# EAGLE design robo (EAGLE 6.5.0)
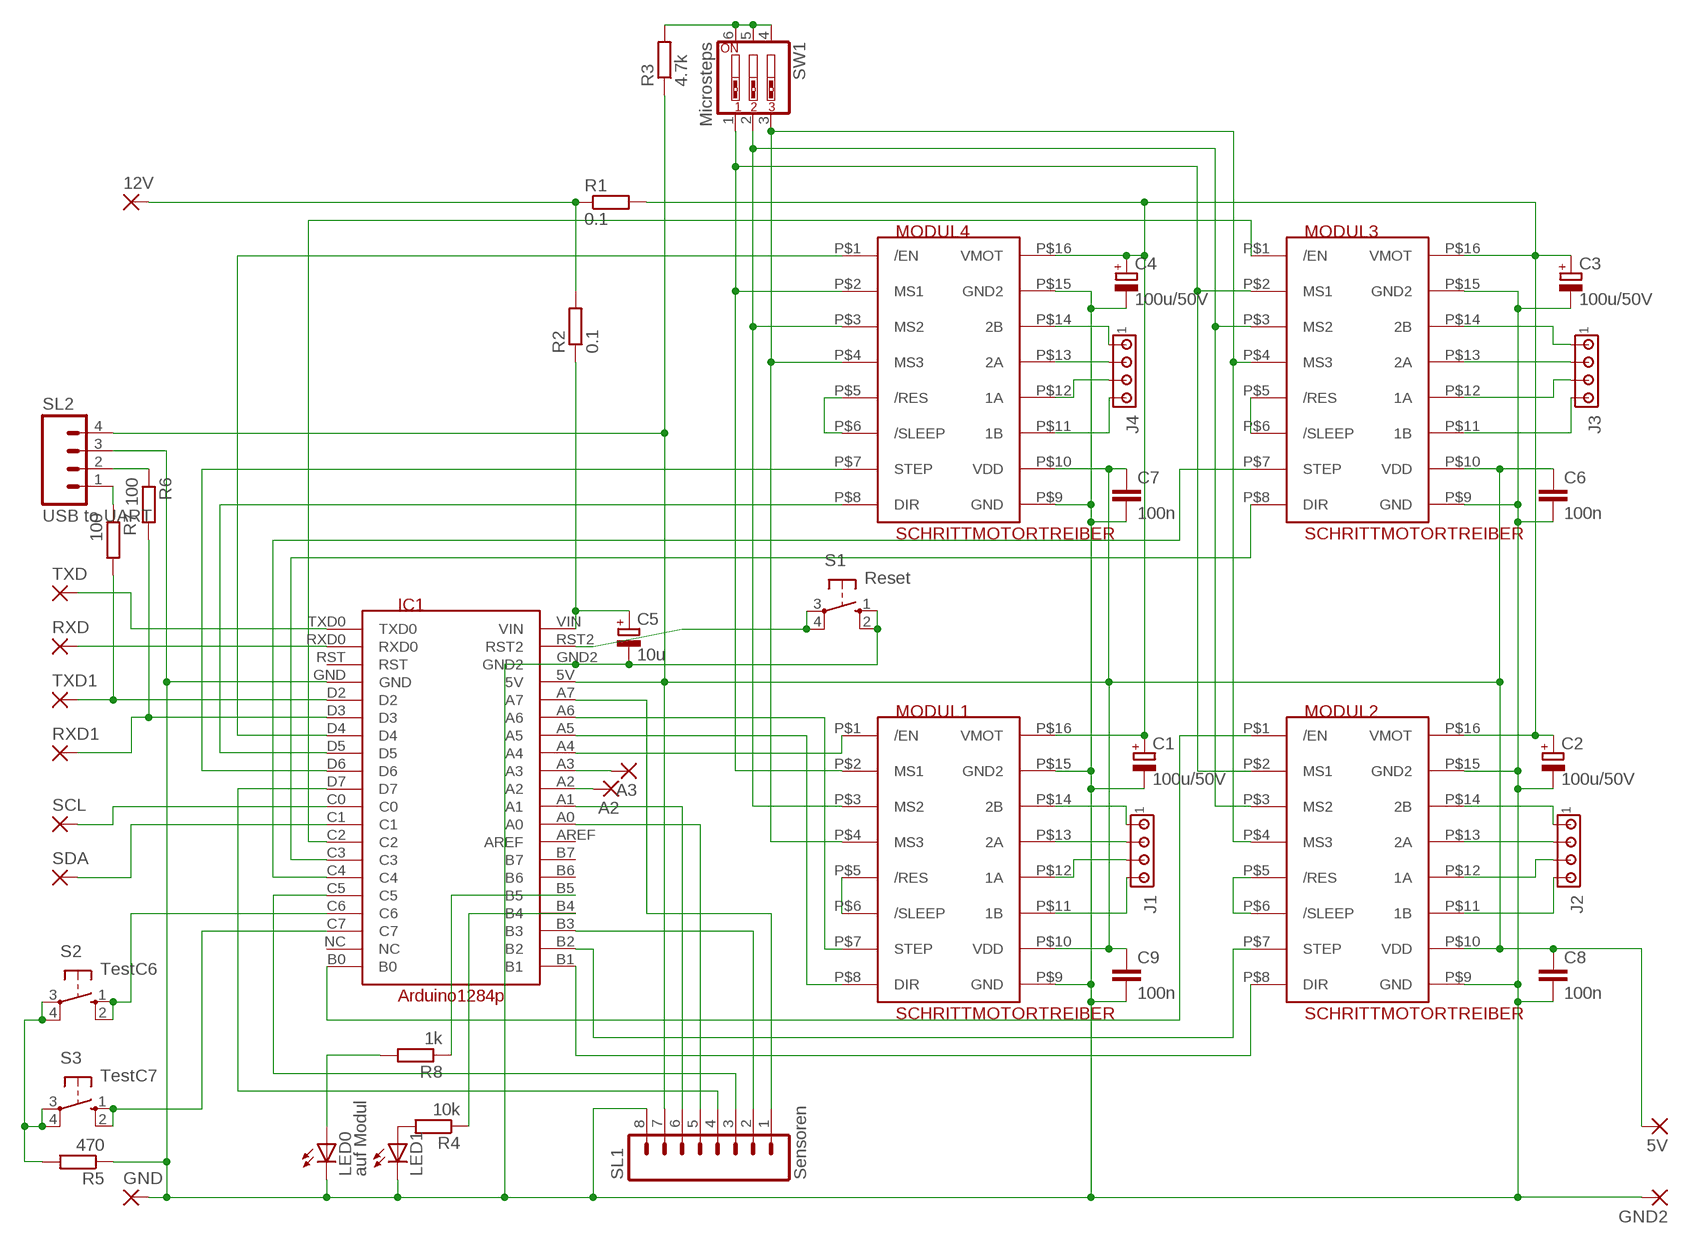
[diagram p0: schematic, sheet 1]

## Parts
5V  WIREPAD2,54/0,9  [2,54/0,9]
12V  WIREPAD3,17/1,1  [3,17/1,1]
A2  WIREPAD2,54/0,9  [2,54/0,9]
A3  WIREPAD2,54/0,9  [2,54/0,9]
C1  100u/50V  CPOL-EUE3.5-8  [E3,5-8]
C2  100u/50V  CPOL-EUE3.5-8  [E3,5-8]
C3  100u/50V  CPOL-EUE3.5-8  [E3,5-8]
C4  100u/50V  CPOL-EUE3.5-8  [E3,5-8]
C5  10u  CPOL-EUE2.5-6  [E2,5-6]
C6  100n  C2,5-3  [C2.5-3]
C7  100n  C2,5-3  [C2.5-3]
C8  100n  C2,5-3  [C2.5-3]
C9  100n  C2,5-3  [C2.5-3]
GND  WIREPAD3,17/1,1  [3,17/1,1]
GND2  WIREPAD2,54/0,9  [2,54/0,9]
IC1  Arduino1284p  ARDUINO1284P  [ARDUINO1284P]
J1  MTA04-100  [10X04MTA]
J2  MTA04-100  [10X04MTA]
J3  MTA04-100  [10X04MTA]
J4  MTA04-100  [10X04MTA]
LED0  auf Modul  LED3MM  [LED3MM]
LED1  LED3MM  [LED3MM]
MODUL1  SCHRITTMOTORTREIBER  [SCHRITTMOTORTREIBER]
MODUL2  SCHRITTMOTORTREIBER  [SCHRITTMOTORTREIBER]
MODUL3  SCHRITTMOTORTREIBER  [SCHRITTMOTORTREIBER]
MODUL4  SCHRITTMOTORTREIBER  [SCHRITTMOTORTREIBER]
R1  0.1  R-EU_0204/7  [0204/7]
R2  0.1  R-EU_0204/7  [0204/7]
R3  4.7k  R-EU_0204/7  [0204/7]
R4  10k  R-EU_0204/7  [0204/7]
R5  470  R-EU_0204/7  [0204/7]
R6  100  R-EU_0207/12  [0207/12]
R7  100  R-EU_0207/12  [0207/12]
R8  1k  R-EU_0204/7  [0204/7]
RXD  WIREPAD2,54/0,9  [2,54/0,9]
RXD1  WIREPAD2,54/0,9  [2,54/0,9]
S1  Reset  10-XX  [B3F-10XX]
S2  TestC6  10-XX  [B3F-10XX]
S3  TestC7  10-XX  [B3F-10XX]
SCL  WIREPAD2,54/0,9  [2,54/0,9]
SDA  WIREPAD2,54/0,9  [2,54/0,9]
SL1  Sensoren  M08  [08P]
SL2  USB to UART  M04  [04P]
SW1  Microsteps  SW_DIP-3  [EDG-03]
TXD  WIREPAD2,54/0,9  [2,54/0,9]
TXD1  WIREPAD2,54/0,9  [2,54/0,9]

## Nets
GND [sehrdick]: C1.- C2.- C3.- C4.- C5.- C6.2 C7.2 C8.2 C9.2 GND2.1(P) GND.1(P) IC1.GND IC1.GND2 LED0.K(C) LED1.K(C) MODUL1.P$9(GND) MODUL1.P$15(GND2) MODUL2.P$9(GND) MODUL2.P$15(GND2) MODUL3.P$9(GND) MODUL3.P$15(GND2) MODUL4.P$9(GND) MODUL4.P$15(GND2) R5.1 S1.1(S) S1.2(S1) SL1.8 SL2.3
N$1 [dick]: J3.1 MODUL3.P$14(2B)
N$2 [dick]: J3.2 MODUL3.P$13(2A)
N$3 [dick]: J3.4 MODUL3.P$11(1B)
N$4: MODUL4.P$5(/RES) MODUL4.P$6(/SLEEP)
N$5: MODUL3.P$5(/RES) MODUL3.P$6(/SLEEP)
N$6: MODUL2.P$5(/RES) MODUL2.P$6(/SLEEP)
N$7: MODUL1.P$5(/RES) MODUL1.P$6(/SLEEP)
N$8 [dick]: J3.3 MODUL3.P$12(1A)
N$9 [dick]: J4.1 MODUL4.P$14(2B)
N$10 [dick]: J4.2 MODUL4.P$13(2A)
N$11 [dick]: J4.4 MODUL4.P$11(1B)
N$12 [dick]: J4.3 MODUL4.P$12(1A)
N$13 [dick]: J1.1 MODUL1.P$14(2B)
N$14 [dick]: J1.2 MODUL1.P$13(2A)
N$15 [dick]: J1.3 MODUL1.P$12(1A)
N$16 [dick]: J1.4 MODUL1.P$11(1B)
N$17 [dick]: J2.1 MODUL2.P$14(2B)
N$18 [dick]: J2.2 MODUL2.P$13(2A)
N$19 [dick]: J2.3 MODUL2.P$12(1A)
N$20 [dick]: J2.4 MODUL2.P$11(1B)
N$21 [sehrdick]: 12V.1(P) R1.1 R2.2
N$22: IC1.A0 SL1.5
N$23: IC1.A5 MODUL1.P$8(DIR)
N$24 [dick]: IC1.RXD0 RXD.1(P)
N$25: MODUL1.P$3(MS2) MODUL2.P$3(MS2) MODUL3.P$3(MS2) MODUL4.P$3(MS2) SW1.2
N$26 [dick]: IC1.TXD0 TXD.1(P)
N$27: MODUL1.P$4(MS3) MODUL2.P$4(MS3) MODUL3.P$4(MS3) MODUL4.P$4(MS3) SW1.3
N$28: R3.2 SW1.4 SW1.5 SW1.6
N$29: MODUL1.P$2(MS1) MODUL2.P$2(MS1) MODUL3.P$2(MS1) MODUL4.P$2(MS1) SW1.1
N$30: IC1.A6 MODUL1.P$7(STEP)
N$31: IC1.A7 SL1.1
N$32: IC1.A4 MODUL1.P$1(/EN)
N$33: IC1.B0 MODUL2.P$1(/EN)
N$34: IC1.B1 MODUL2.P$8(DIR)
N$35: IC1.B2 MODUL2.P$7(STEP)
N$36: IC1.B3 SL1.2
N$37: IC1.C2 MODUL3.P$1(/EN)
N$38: IC1.C3 MODUL3.P$8(DIR)
N$39: IC1.C4 MODUL3.P$7(STEP)
N$40: IC1.C5 SL1.3
N$41: IC1.D4 MODUL4.P$1(/EN)
N$42: IC1.D5 MODUL4.P$8(DIR)
N$43: IC1.D6 MODUL4.P$7(STEP)
N$44: IC1.D7 SL1.4
N$45 [dick]: IC1.D2 R7.2 TXD1.1(P)
N$46 [dick]: IC1.D3 R6.2 RXD1.1(P)
N$47: IC1.A1 SL1.6
N$48: IC1.RST2 S1.3(P) S1.4(P1)
N$49: IC1.C0 SCL.1(P)
N$50: IC1.C1 SDA.1(P)
N$51: A2.1(P) IC1.A2
N$52: A3.1(P) IC1.A3
N$53: LED1.A R4.2
N$54: IC1.B4 R4.1
N$55: IC1.C6 S2.1(S) S2.2(S1)
N$56: IC1.C7 S3.1(S) S3.2(S1)
N$57: R5.2 S2.3(P) S2.4(P1) S3.3(P) S3.4(P1)
N$58 [dick]: R7.1 SL2.1
N$59 [dick]: R6.1 SL2.2
N$60: LED0.A R8.2
N$61: IC1.B5 R8.1
VDD [dick]: 5V.1(P) C6.1 C7.1 C8.1 C9.1 IC1.5V MODUL1.P$10(VDD) MODUL2.P$10(VDD) MODUL3.P$10(VDD) MODUL4.P$10(VDD) R3.1 SL1.7 SL2.4
VIN [dick]: C5.+ IC1.VIN R2.1
VMOT [sehrdick]: C1.+ C2.+ C3.+ C4.+ MODUL1.P$16(VMOT) MODUL2.P$16(VMOT) MODUL3.P$16(VMOT) MODUL4.P$16(VMOT) R1.2
Unconnected: IC1.AREF IC1.B6 IC1.B7 IC1.NC IC1.RST

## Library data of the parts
5V 12V A2 A3 GND GND2 RXD RXD1 SCL SDA TXD TXD1 = wirepad:WIREPAD: Wire PAD connect wire on PCB
C1-C5 = rcl:CPOL-EU: POLARIZED CAPACITOR, European symbol
C6-C9 = capacitor-wima:C: CAPACITOR
IC1 = arduino:ARDUINO1284P
J1-J4 = con-amp:MTA04-100: AMP connector
LED0 LED1 = led:LED: LED
MODUL1-MODUL4 = arduino:SCHRITTMOTORTREIBER
R1-R8 = rcl:R-EU_: RESISTOR, European symbol
S1-S3 = switch-omron:10-XX: OMRON SWITCH; MPN: B3F-1000; OC_FARNELL: 176432; OC_NEWARK: 36M3542
SL1 = con-amp-quick:M08: AMP QUICK CONNECTOR; OC_FARNELL: unknown; OC_NEWARK: unknown
SL2 = con-amp-quick:M04: AMP QUICK CONNECTOR; OC_FARNELL: unknown; OC_NEWARK: unknown
SW1 = special:SW_DIP-3: DIP SWITCH

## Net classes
0 default: width 0.508 mm
1 dick: width 0.762 mm
2 sehrdick: width 1.27 mm

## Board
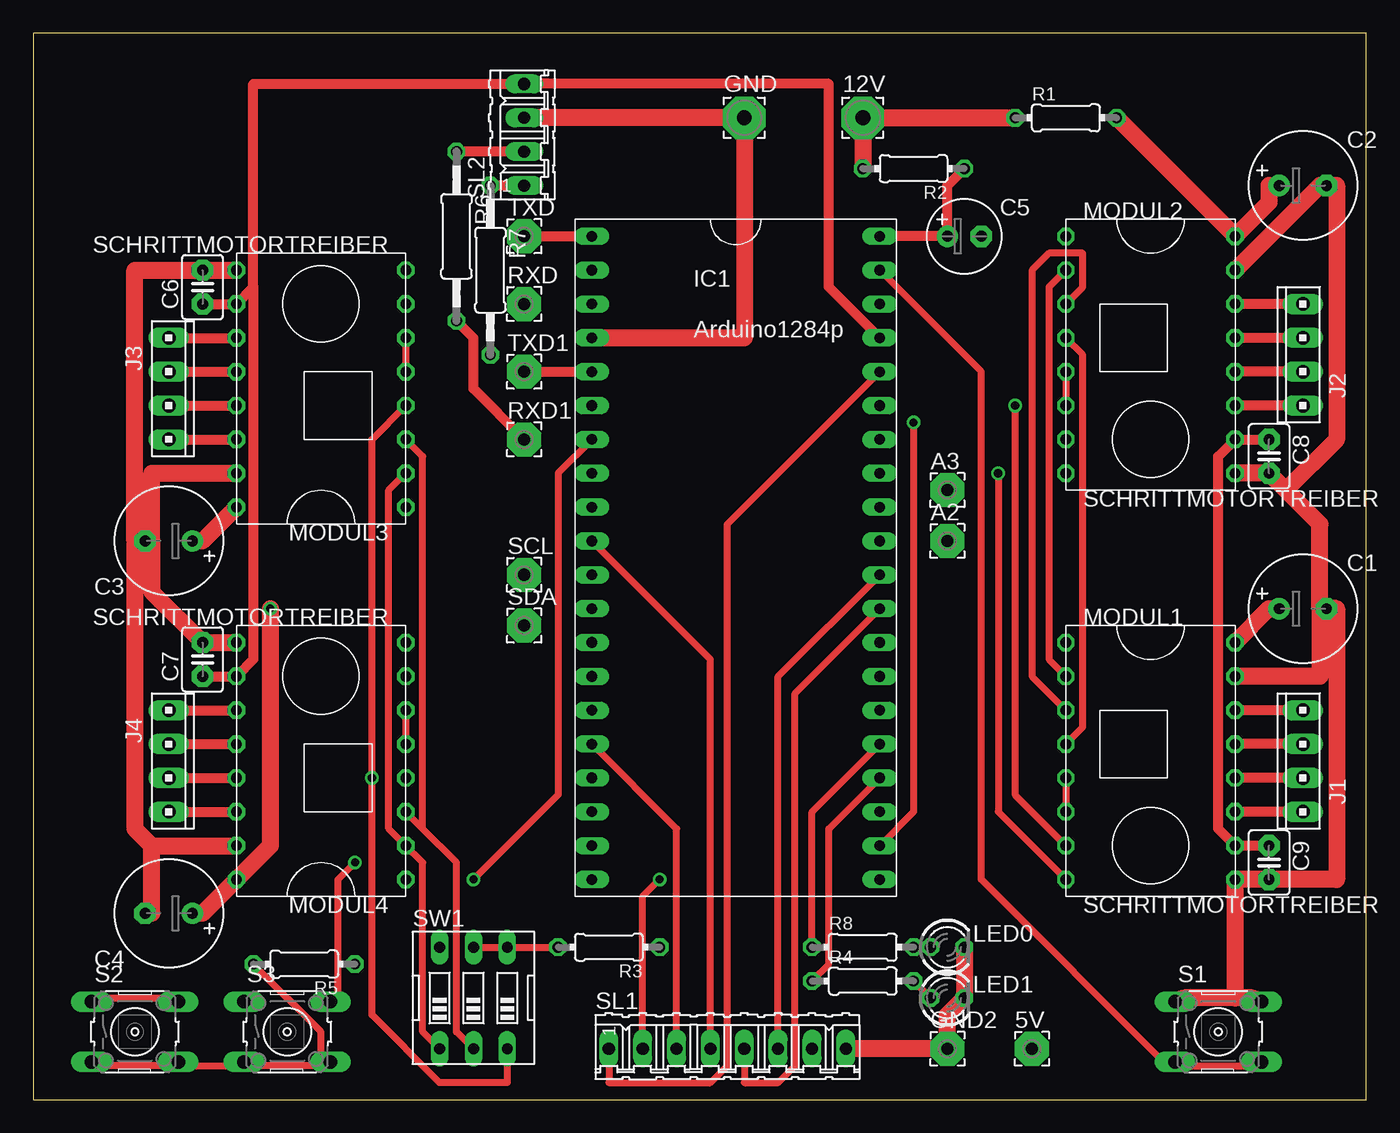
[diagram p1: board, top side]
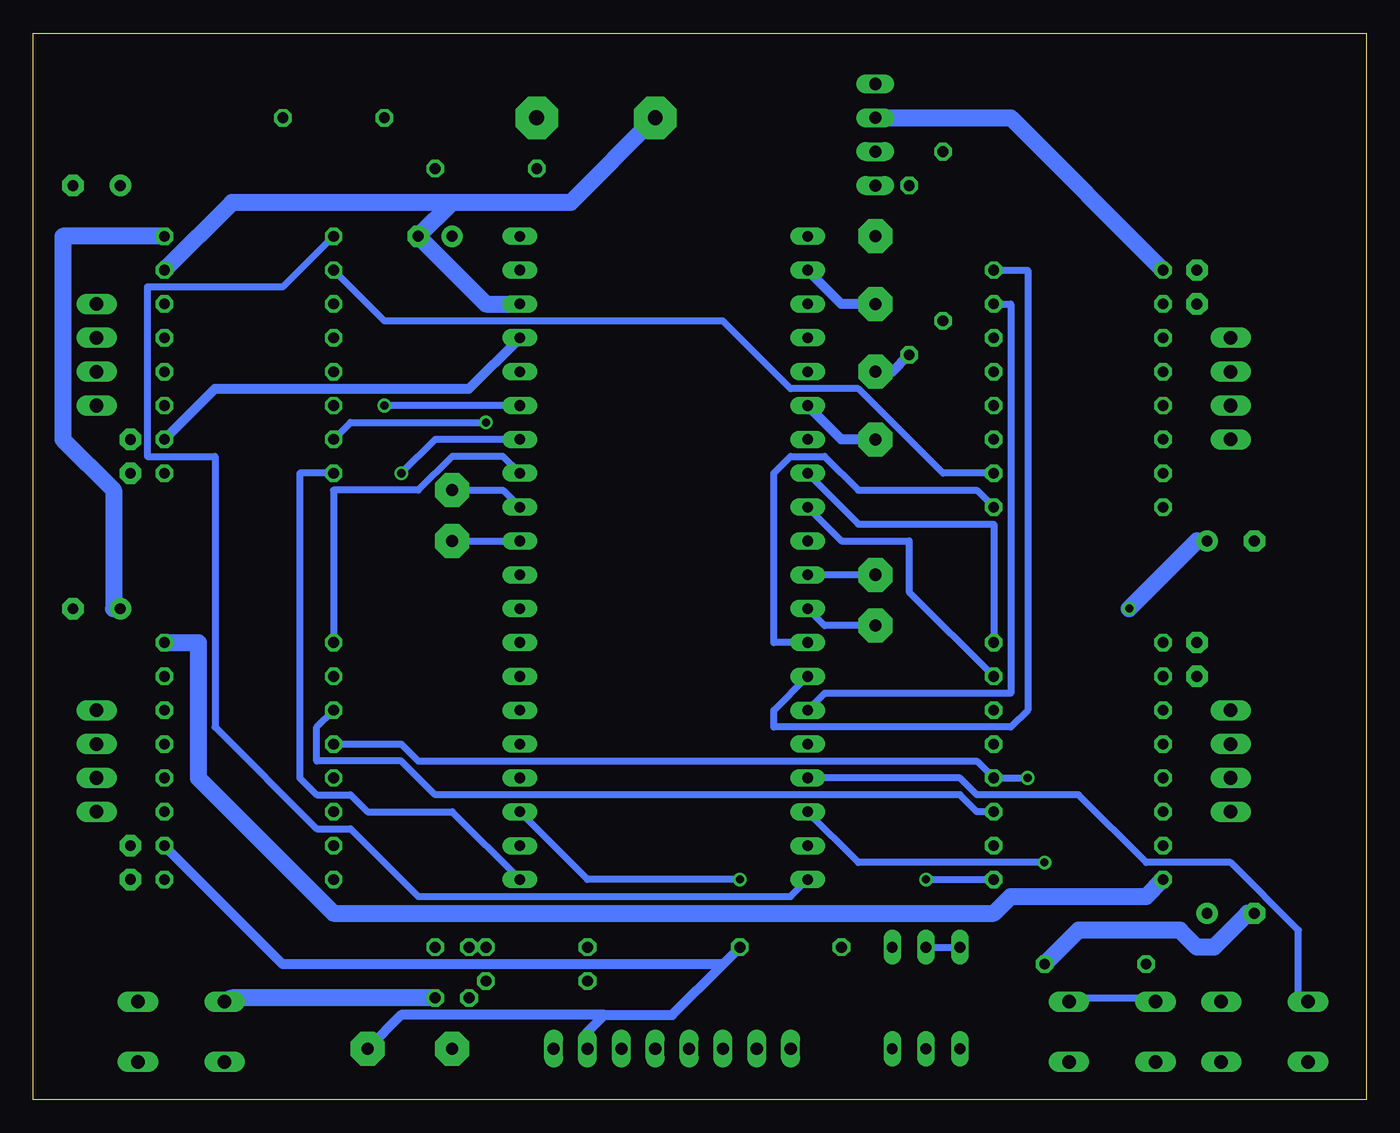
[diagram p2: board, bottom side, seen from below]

Size 100 x 80 mm. Coordinates in mm from the lower left corner, seen from the top.
Outline: 0,0 100,0 100,80 0,80 0,0
Copper layers (1*16): Top 0.035mm / dielectric 1.5mm / Bottom 0.035mm
Design rules "default": minimum track width 10mil, minimum drill 24mil, track to track 8mil, track to pad 8mil, pad to pad 8mil, via to via 8mil, smd to smd 8mil, copper to edge 40mil, drill to drill 8mil, minimum pad ring 10mil, minimum via ring 8mil, stop-mask expansion 4mil, vias tented up to drill 0mil, thermal gap 10mil

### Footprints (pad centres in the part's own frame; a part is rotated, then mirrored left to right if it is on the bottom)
2,54/0,9 = drill 0.914 pad 2.54 octagon: 1 0,0
3,17/1,1 = drill 1.118 pad 3.175 octagon: 1 0,0
E3,5-8 = drill 0.813 pad 1.6: + -1.778,0 | drill 0.813 pad 1.6 octagon: - 1.778,0
E2,5-6 = drill 0.813 pad 1.6: + -1.27,0 | drill 0.813 pad 1.6 octagon: - 1.27,0
C2.5-3 = drill 0.813 pad 1.6 octagon: 1 -1.27,0; 2 1.27,0
ARDUINO1284P = drill 0.8 long: 5V 10.16,3.81; A0 10.16,-16.51; A1 10.16,-13.97; A2 10.16,-11.43; A3 10.16,-8.89; A4 10.16,-6.35; A5 10.16,-3.81; A6 10.16,-1.27; A7 10.16,1.27; AREF 10.16,-19.05; B0 -11.43,-36.83; B1 10.16,-36.83; B2 10.16,-34.29; B3 10.16,-31.75; B4 10.16,-29.21; B5 10.16,-26.67; B6 10.16,-24.13; B7 10.16,-21.59; C0 -11.43,-13.97; C1 -11.43,-16.51; C2 -11.43,-19.05; C3 -11.43,-21.59; C4 -11.43,-24.13; C5 -11.43,-26.67; C6 -11.43,-29.21; C7 -11.43,-31.75; D2 -11.43,1.27; D3 -11.43,-1.27; D4 -11.43,-3.81; D5 -11.43,-6.35; D6 -11.43,-8.89; D7 -11.43,-11.43; GND -11.43,3.81; GND2 10.16,6.35; NC -11.43,-34.29; RST -11.43,6.35; RST2 10.16,8.89; RXD0 -11.43,8.89; TXD0 -11.43,11.43; VIN 10.16,11.43
10X04MTA = drill 1.016 long: 1 3.81,0; 2 1.27,0; 3 -1.27,0; 4 -3.81,0
LED3MM = drill 0.813 octagon: A -1.27,0; K 1.27,0
SCHRITTMOTORTREIBER = drill 0.8 octagon: P$1 -6.35,8.89; P$2 -6.35,6.35; P$3 -6.35,3.81; P$4 -6.35,1.27; P$5 -6.35,-1.27; P$6 -6.35,-3.81; P$7 -6.35,-6.35; P$8 -6.35,-8.89; P$9 6.35,-8.89; P$10 6.35,-6.35; P$11 6.35,-3.81; P$12 6.35,-1.27; P$13 6.35,1.27; P$14 6.35,3.81; P$15 6.35,6.35; P$16 6.35,8.89
0204/7 = drill 0.813 octagon: 1 -3.81,0; 2 3.81,0
0207/12 = drill 0.813 octagon: 1 -6.35,0; 2 6.35,0
B3F-10XX = drill 1.016 long: 1 -3.251,2.261; 2 3.251,2.261; 3 -3.251,-2.261; 4 3.251,-2.261
08P = drill 0.914 long: 1 -8.89,0; 2 -6.35,0; 3 -3.81,0; 4 -1.27,0; 5 1.27,0; 6 3.81,0; 7 6.35,0; 8 8.89,0
04P = drill 0.914 long: 1 -3.81,0; 2 -1.27,0; 3 1.27,0; 4 3.81,0
EDG-03 = drill 0.813 long: 1 -2.54,-3.81; 2 0,-3.81; 3 2.54,-3.81; 4 2.54,3.81; 5 0,3.81; 6 -2.54,3.81

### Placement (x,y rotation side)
5V  74.93,3.81 0 top
12V  62.23,73.66 0 top
A2  68.58,41.91 0 top
A3  68.58,45.72 0 top
C1  95.25,36.83 0 top
C2  95.25,68.58 0 top
C3  10.16,41.91 180 top
C4  10.16,13.97 180 top
C5  69.85,64.77 0 top
C6  12.7,60.96 90 top
C7  12.7,33.02 90 top
C8  92.71,48.26 270 top
C9  92.71,17.78 270 top
GND  53.34,73.66 0 top
GND2  68.58,3.81 0 top
IC1  53.34,53.34 0 top
J1  95.25,25.4 90 top
J2  95.25,55.88 90 top
J3  10.16,53.34 270 top
J4  10.16,25.4 270 top
LED0  68.58,11.43 0 top
LED1  68.58,7.62 0 top
MODUL1  83.82,25.4 0 top
MODUL2  83.82,55.88 0 top
MODUL3  21.59,53.34 180 top
MODUL4  21.59,25.4 180 top
R1  77.47,73.66 0 top
R2  66.04,69.85 180 top
R3  43.18,11.43 180 top
R4  62.23,8.89 0 top
R5  20.32,10.16 180 top
R6  31.75,64.77 270 top
R7  34.29,62.23 270 top
R8  62.23,11.43 0 top
RXD  36.83,59.69 0 top
RXD1  36.83,49.53 0 top
S1  88.9,5.08 0 top
S2  7.62,5.08 0 top
S3  19.05,5.08 0 top
SCL  36.83,39.37 0 top
SDA  36.83,35.56 0 top
SL1  52.07,3.81 0 top
SL2  36.83,72.39 90 top
SW1  33.02,7.62 0 top
TXD  36.83,64.77 0 top
TXD1  36.83,54.61 0 top

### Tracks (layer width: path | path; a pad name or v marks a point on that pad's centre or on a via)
GND
  Top 1.27: 8.89,19.05 MODUL4.P$15 | 8.89,19.05 8.89,13.97 C4.- | MODUL3.P$9 C6.2 7.62,62.23 7.62,41.91 | MODUL4.P$9 C7.2 8.89,38.1 8.89,41.91 | MODUL3.P$15 8.89,46.99 8.89,41.91 | 8.89,41.91 C3.- 7.62,41.91 | 8.89,19.05 7.62,20.32 7.62,41.91 | 90.17,7.62 91.44,7.62 S1.2 | 90.17,7.62 86.36,7.62 S1.1 | 90.17,7.62 MODUL1.P$9 C9.2 97.79,16.51 97.79,36.83 C1.- 96.52,36.83 | LED0.K LED1.K 68.58,6.35 GND2.1 SL1.8 | MODUL2.P$9 C8.2 93.98,45.72 | MODUL1.P$15 96.52,31.75 96.52,36.83 | 93.98,45.72 96.52,43.18 96.52,36.83 | MODUL2.P$15 96.52,68.58 C2.- 97.79,68.58 97.79,49.53 93.98,45.72 | IC1.GND 53.34,57.15 GND.1 SL2.3
  Bottom 1.27: R5.1 21.59,12.7 13.97,12.7 12.7,11.43 11.43,11.43 8.89,13.97 C4.- | LED1.K 85.09,7.62 S1.1 | IC1.GND2 66.04,59.69 C5.- 68.58,67.31 | 68.58,67.31 59.69,67.31 GND.1 | MODUL2.P$15 85.09,67.31 68.58,67.31 | MODUL3.P$9 26.67,73.66 SL2.3
N$1
  Top 0.762: J3.1 MODUL3.P$14
N$2
  Top 0.762: J3.2 MODUL3.P$13
N$3
  Top 0.762: J3.4 MODUL3.P$11
N$4
  Top 0.508: MODUL4.P$6 MODUL4.P$5
N$5
  Top 0.508: MODUL3.P$6 MODUL3.P$5
N$6
  Top 0.508: MODUL2.P$5 MODUL2.P$6
N$7
  Top 0.508: MODUL1.P$5 MODUL1.P$6
N$8
  Top 0.762: J3.3 MODUL3.P$12
N$9
  Top 0.762: J4.1 MODUL4.P$14
N$10
  Top 0.762: J4.2 MODUL4.P$13
N$11
  Top 0.762: J4.4 MODUL4.P$11
N$12
  Top 0.762: J4.3 MODUL4.P$12
N$13
  Top 0.762: J1.1 MODUL1.P$14
N$14
  Top 0.762: J1.2 MODUL1.P$13
N$15
  Top 0.762: J1.3 MODUL1.P$12
N$16
  Top 0.762: J1.4 MODUL1.P$11
N$17
  Top 0.762: J2.1 MODUL2.P$14
N$18
  Top 0.762: J2.2 MODUL2.P$13
N$19
  Top 0.762: J2.3 MODUL2.P$12
N$20
  Top 0.762: J2.4 MODUL2.P$11
N$21
  Top 1.27: R2.2 12V.1 R1.1
N$22
  Top 0.508: IC1.A0 57.15,30.48 57.15,2.54 55.88,1.27 53.34,1.27 SL1.5
N$23  (via drill 0.61)
  Top 0.508: MODUL1.P$8 72.39,21.59 v72.39,46.99
  Bottom 0.508: v72.39,46.99 69.85,49.53 IC1.A5
N$24
  Bottom 0.762: IC1.RXD0 39.37,59.69 RXD.1
N$25
  Top 0.508: MODUL1.P$3 74.93,31.75 74.93,62.23 76.2,63.5 78.74,63.5 78.74,60.96 MODUL2.P$3 | 29.21,20.32 31.75,17.78 31.75,5.08 SW1.2 | 29.21,20.32 MODUL4.P$3 | MODUL3.P$3 29.21,48.26 29.21,20.32
  Bottom 0.508: MODUL1.P$3 78.74,27.94 78.74,25.4 72.39,25.4 69.85,22.86 30.48,22.86 29.21,21.59 MODUL4.P$3
N$26
  Top 0.762: TXD.1 IC1.TXD0
N$27  (via drill 0.61)
  Top 0.508: MODUL3.P$4 25.4,49.53 v25.4,24.13 25.4,6.35 30.48,1.27 35.56,1.27 SW1.3 | MODUL2.P$4 78.74,55.88 78.74,27.94 MODUL1.P$4
  Bottom 0.508: MODUL1.P$4 72.39,26.67 71.12,25.4 29.21,25.4 MODUL4.P$4 v25.4,24.13
N$28
  Top 0.508: SW1.5 SW1.4 R3.2
  Bottom 0.508: SW1.5 SW1.6
N$29
  Top 0.508: MODUL1.P$2 76.2,33.02 76.2,60.96 MODUL2.P$2 | SW1.1 29.21,5.08 29.21,17.78 MODUL4.P$2 26.67,20.32 26.67,45.72 MODUL3.P$2
  Bottom 0.508: MODUL2.P$2 73.66,58.42 48.26,58.42 43.18,53.34 38.1,53.34 31.75,46.99 MODUL3.P$2
N$30  (via drill 0.61)
  Top 0.508: MODUL1.P$7 73.66,22.86 v73.66,52.07
  Bottom 0.508: IC1.A6 v73.66,52.07
N$31
  Top 0.508: IC1.A7 52.07,43.18 52.07,2.54 50.8,1.27 43.18,1.27 SL1.1
N$32
  Bottom 0.508: MODUL1.P$1 77.47,45.72 71.12,45.72 68.58,48.26 64.77,48.26 IC1.A4
N$33
  Bottom 0.508: IC1.B0 43.18,15.24 71.12,15.24 76.2,20.32 78.74,20.32 86.36,27.94 86.36,48.26 91.44,48.26 91.44,60.96 81.28,60.96 MODUL2.P$1
N$34
  Bottom 0.508: IC1.B1 68.58,21.59 74.93,21.59 76.2,22.86 78.74,22.86 80.01,24.13 80.01,46.99 MODUL2.P$8
N$35  (via drill 0.61)
  Top 0.508: IC1.B2 66.04,21.59 v66.04,50.8
  Bottom 0.508: v66.04,50.8 76.2,50.8 MODUL2.P$7
N$36  (via drill 0.61)
  Top 0.508: v46.99,16.51 45.72,15.24 SL1.2
  Bottom 0.508: IC1.B3 58.42,16.51 v46.99,16.51
N$37
  Bottom 0.508: MODUL3.P$1 29.21,45.72 38.1,45.72 40.64,48.26 43.18,48.26 44.45,46.99 44.45,34.29 IC1.C2
N$38
  Bottom 0.508: IC1.C3 44.45,29.21 44.45,27.94 26.67,27.94 25.4,29.21 25.4,62.23 MODUL3.P$8
N$39
  Bottom 0.508: IC1.C4 40.64,30.48 26.67,30.48 26.67,59.69 MODUL3.P$7
N$40
  Top 0.508: IC1.C5 48.26,20.32 SL1.3
N$41  (via drill 0.61)
  Top 0.508: v33.02,16.51 39.37,22.86 39.37,46.99 IC1.D4
  Bottom 0.508: v33.02,16.51 MODUL4.P$1
N$42
  Bottom 0.508: MODUL4.P$8 27.94,43.18 38.1,43.18 IC1.D5
N$43
  Bottom 0.508: MODUL4.P$7 34.29,38.1 34.29,41.91 39.37,41.91 IC1.D6
N$44
  Top 0.508: IC1.D7 50.8,33.02 SL1.4
N$45
  Top 0.762: TXD1.1 IC1.D2
  Bottom 0.762: R7.2 35.56,54.61 TXD1.1
N$46
  Top 0.762: R6.2 33.02,57.15 33.02,53.34 RXD1.1
  Bottom 0.762: IC1.D3 39.37,49.53 RXD1.1
N$47
  Top 0.508: IC1.A1 55.88,31.75 SL1.6
N$48
  Top 0.508: IC1.RST2 71.12,54.61 71.12,16.51 85.09,2.54 S1.3 86.36,2.54 91.44,2.54 S1.4
N$49
  Bottom 0.508: SCL.1 IC1.C0
N$50
  Bottom 0.508: IC1.C1 40.64,35.56 SDA.1
N$51
  Bottom 0.508: A2.1 IC1.A2
N$52
  Bottom 0.508: IC1.A3 64.77,45.72 A3.1
N$53
  Top 0.508: LED1.A R4.2
N$54
  Top 0.508: IC1.B4 59.69,20.32 59.69,10.16 R4.1
N$55
  Top 0.508: S2.2 10.16,7.62 5.08,7.62 S2.1
  Bottom 0.508: IC1.C6 30.48,24.13 29.21,22.86 21.59,22.86 16.51,17.78 10.16,17.78 5.08,12.7 5.08,7.62 S2.1
N$56  (via drill 0.61)
  Top 0.508: v24.13,17.78 22.86,16.51 22.86,7.62 S3.2
  Bottom 0.508: IC1.C7 38.1,17.78 v24.13,17.78 | S3.1 16.51,7.62 21.59,7.62 S3.2
N$57
  Top 0.508: S2.3 5.08,2.54 10.16,2.54 S2.4 11.43,2.54 15.24,2.54 S3.3 16.51,2.54 21.59,2.54 | R5.2 21.59,5.08 21.59,2.54 | 21.59,2.54 S3.4
N$58
  Top 0.762: SL2.1 R7.1
N$59
  Top 0.762: SL2.2 R6.1
N$60
  Top 0.508: LED0.A R8.2
N$61
  Top 0.508: IC1.B5 58.42,21.59 R8.1
VDD
  Top 0.762: C7.1 MODUL4.P$10 16.51,33.02 16.51,60.96 | C6.1 MODUL3.P$10 16.51,60.96 | 16.51,60.96 16.51,76.2 SL2.4 59.69,76.2 59.69,60.96 IC1.5V | C8.1 MODUL2.P$10 88.9,48.26 88.9,20.32 MODUL1.P$10 C9.1
  Bottom 0.762: IC1.5V 67.31,53.34 86.36,53.34 MODUL2.P$10 | 48.26,10.16 52.07,6.35 57.15,6.35 | 48.26,10.16 R3.1 | 57.15,6.35 58.42,5.08 SL1.7 | MODUL1.P$10 81.28,10.16 48.26,10.16 | 5V.1 72.39,6.35 57.15,6.35
VIN
  Top 0.762: IC1.VIN C5.+ 68.58,68.58 R2.1
VMOT  (via drill 0.61)
  Top 1.27: C4.+ 12.7,13.97 MODUL4.P$16 17.78,19.05 v17.78,36.83 | MODUL3.P$16 12.7,41.91 C3.+ | MODUL1.P$16 92.71,36.83 C1.+ | C2.+ 92.71,68.58 92.71,67.31 MODUL2.P$16 R1.2
  Bottom 1.27: v17.78,36.83 12.7,41.91 C3.+ | MODUL2.P$16 97.79,64.77 97.79,49.53 93.98,45.72 93.98,36.83 C1.+ | MODUL4.P$16 16.51,15.24 26.67,15.24 27.94,13.97 77.47,13.97 87.63,24.13 87.63,34.29 MODUL1.P$16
